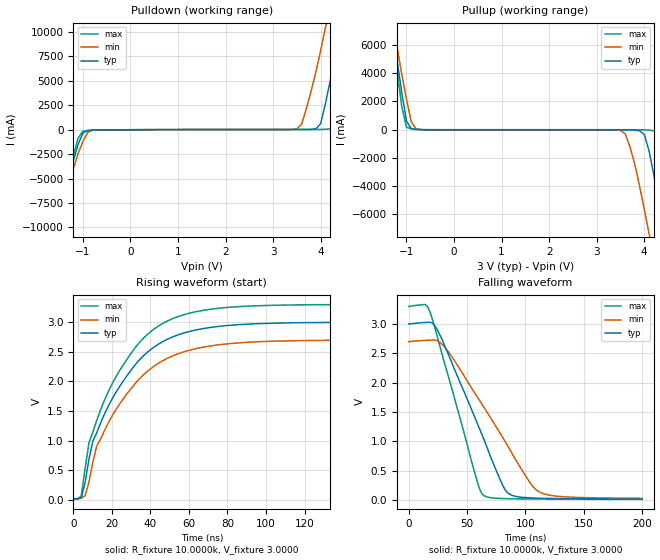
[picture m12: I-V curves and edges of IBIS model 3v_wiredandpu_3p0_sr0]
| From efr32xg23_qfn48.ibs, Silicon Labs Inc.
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|   Model 3v_wiredandpu_3p0_sr0
[Model]  3v_wiredandpu_3p0_sr0
Model_type Output
Polarity   Inverting
Enable   Active-Low
C_comp   1.6300pF   1.4000pF   2.7000pF
[Temperature Range]   25.0000   0.1250k   -40.0000
[Pullup Reference]   3.0000V   2.7000V   3.3000V
[Pulldown Reference]   0.0V   0.0V   0.0V
[POWER Clamp Reference]   3.0000V   2.7000V   3.3000V
[GND Clamp Reference]   0.0V   0.0V   0.0V
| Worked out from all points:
|   slope of the pulldown table from 0 to 0.45 V, typ, clamps not added: 51.6 ohm
|   slope of the pullup table from 0 to 0.45 V, typ, clamps not added: 44.4 kohm
|   rising waveform, R_fixture 10.0000k, V_fixture 3.0000: 20-80 % time 27.8ns typ, 28.6ns min, 27.2ns max; typ from 0.013 V to 3 V
|   falling waveform, R_fixture 10.0000k, V_fixture 3.0000: 20-80 % time 37.1ns typ, 49.5ns min, 27.2ns max; typ from 3 V to 0.014 V
[Pulldown]
|Voltage   I(typ)   I(min)   I(max)
-3V       -32.58A    -30.59A    -34.3A
-1.6V     -10.63A    -10.8A     -10.6A
-1V       -332.6mA   -1.21A     -150.8mA
-700mV    -19.14mA   -16.32mA   -23.31mA
3.5V      19.25mA    78.91mA    25.55mA
3.7V      24.82mA    2.187A     25.57mA
4V        632.8mA    8.108A     32.07mA
4.1V      2.678A     10.43A     48.62mA
4.3V      7.523A     15.18A     198.8mA
4.4V      10.19A     17.49A     1.688A
4.7V      18.29A     24.05A     10.15A
6V        48.89A     49.41A     46.12A
[Pullup]
|Voltage   I(typ)   I(min)   I(max)
-3V       48.87A     43.59A     53.88A
-1.3V     7.504A     8.096A     7.139A
-1V       614.1mA    2.175A     173.2mA
-700mV    6.165mA    10.06mA    6.512mA
3.5V      -793uA     -46.9mA    -91.34uA
3.7V      -7.536mA   -1.208A    -137.9uA
4V        -326.3mA   -5.611A    -8.337mA
4.1V      -1.482A    -7.329A    -28.82mA
4.3V      -4.973A    -10.8A     -136.8mA
4.4V      -6.846A    -12.49A    -837.2mA
4.8V      -14.25A    -18.59A    -8.585A
6V        -32.58A    -34.37A    -29.65A
[Ramp]
| variable   typ   min   max
dV/dt_r  0.3310/16.4957n   0.2657/17.6467n   0.4098/15.6310n
dV/dt_f  1.7917/37.0599n   1.6037/49.5130n   1.9737/27.2337n
R_load = 10.0000k
[Rising Waveform]
R_fixture= 10.0000k
V_fixture= 3.0000
V_fixture_min= 2.7000
V_fixture_max= 3.3000
|time   V(typ)   V(min)   V(max)
0s        12.75mV    17.61mV    10.35mV
4.04ns    25.81mV    26.63mV    59.13mV
6.061ns   286mV      65.89mV    526.1mV
8.081ns   687.4mV    300.7mV    958.8mV
10.1ns    987.9mV    637.4mV    1.143V
20.2ns    1.709V     1.421V     1.963V
34.34ns   2.365V     2.045V     2.66V
48.48ns   2.707V     2.385V     3.015V
88.89ns   2.965V     2.658V     3.269V
200ns     3V         2.699V     3.3V
[Falling Waveform]
R_fixture= 10.0000k
V_fixture= 3.0000
V_fixture_min= 2.7000
V_fixture_max= 3.3000
|time   V(typ)   V(min)   V(max)
0s        3V         2.7V       3.3V
14.14ns   3.027V     2.721V     3.333V
18.18ns   3.031V     2.725V     3.212V
24.24ns   2.913V     2.72V      2.809V
32.32ns   2.564V     2.572V     2.225V
58.59ns   1.318V     1.764V     328.8mV
64.65ns   1.025V     1.576V     71.51mV
84.85ns   120.5mV    923.7mV    21.68mV
111.1ns   29.99mV    146.5mV    15.94mV
200ns     13.78mV    27.07mV    10.47mV
